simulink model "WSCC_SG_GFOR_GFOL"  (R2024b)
settings: Solver=ode1  StartTime=0.0  StopTime=sim_config.Tsim  RelTol=1e-3
undefined symbols (not defined in the file or in its folder): sim_config
libraries: myLibrary x24, spsThreePhaseVIMeasurementLib x12, spsPower3phInstantaneousLib x6, spspowerguiLib x1

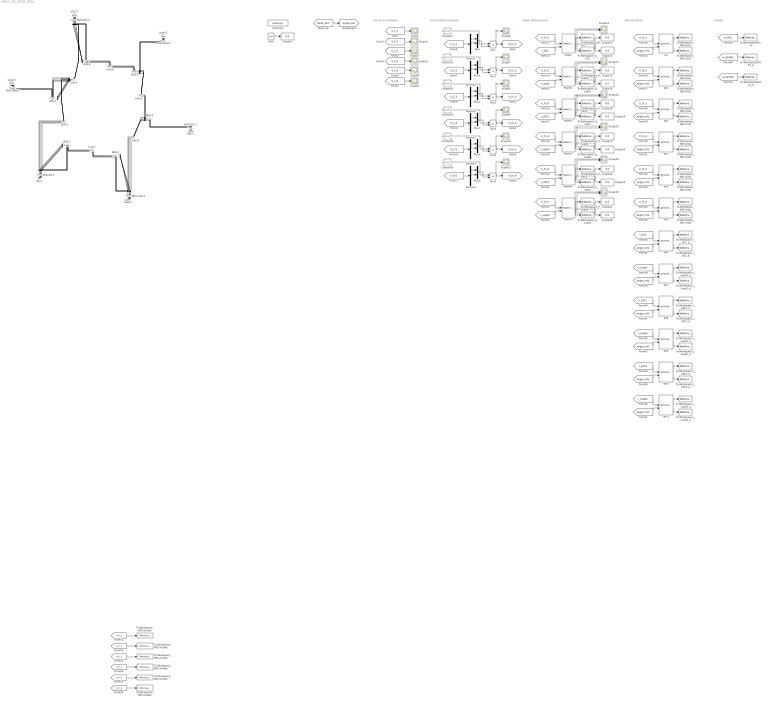
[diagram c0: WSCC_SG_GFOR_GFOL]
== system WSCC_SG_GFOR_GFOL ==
  note: Line-to-Line Voltages
  note: Line-to-Neutral Voltages
  note: Power Measurements
  note: qd0 transforms
  note: omega
  BUS-1 : spsThreePhaseVIMeasurementLib/Three-Phase V-I Measurement  VoltageMeasurement=phase-to-phase  SetLabelV=on  LabelV=V_ll_1  Vpu=off  VpuLL=off  CurrentMeasurement=yes  SetLabelI=on  LabelI=I_1  Ipu=off  Pbase=100e6  Vbase=500e3  OutputType=Complex  PhasorSimulation=off  PSBequivalent=0
  BUS-2 : spsThreePhaseVIMeasurementLib/Three-Phase V-I Measurement  VoltageMeasurement=phase-to-phase  SetLabelV=on  LabelV=V_ll_2  Vpu=off  VpuLL=off  CurrentMeasurement=yes  SetLabelI=on  LabelI=I_2  Ipu=off  Pbase=100e6  Vbase=500e3  OutputType=Complex  PhasorSimulation=off  PSBequivalent=0
  BUS-3 : spsThreePhaseVIMeasurementLib/Three-Phase V-I Measurement  VoltageMeasurement=phase-to-phase  SetLabelV=on  LabelV=V_ll_3  Vpu=off  VpuLL=off  CurrentMeasurement=yes  SetLabelI=on  LabelI=I_3  Ipu=off  Pbase=100e6  Vbase=500e3  OutputType=Complex  PhasorSimulation=off  PSBequivalent=0
  BUS-4 : spsThreePhaseVIMeasurementLib/Three-Phase V-I Measurement  VoltageMeasurement=phase-to-phase  SetLabelV=on  LabelV=V_ll_4  Vpu=off  VpuLL=off  CurrentMeasurement=yes  SetLabelI=on  LabelI=I_4  Ipu=off  Pbase=100e6  Vbase=500e3  OutputType=Complex  PhasorSimulation=off  PSBequivalent=0
  BUS-5 : spsThreePhaseVIMeasurementLib/Three-Phase V-I Measurement  VoltageMeasurement=phase-to-phase  SetLabelV=on  LabelV=V_ll_5  Vpu=off  VpuLL=off  CurrentMeasurement=yes  SetLabelI=on  LabelI=I_5  Ipu=off  Pbase=100e6  Vbase=500e3  OutputType=Complex  PhasorSimulation=off  PSBequivalent=0
  BUS-6 : spsThreePhaseVIMeasurementLib/Three-Phase V-I Measurement  VoltageMeasurement=phase-to-phase  SetLabelV=on  LabelV=V_ll_6  Vpu=off  VpuLL=off  CurrentMeasurement=yes  SetLabelI=on  LabelI=I_6  Ipu=off  Pbase=100e6  Vbase=500e3  OutputType=Complex  PhasorSimulation=off  PSBequivalent=0
  BUS-Load-1 : spsThreePhaseVIMeasurementLib/Three-Phase V-I Measurement  VoltageMeasurement=phase-to-phase  SetLabelV=on  LabelV=V_Load_1  Vpu=off  VpuLL=off  CurrentMeasurement=yes  SetLabelI=on  LabelI=I_Load1  Ipu=off  Pbase=100e6  Vbase=500e3  OutputType=Complex  PhasorSimulation=off  PSBequivalent=0
  BUS-Load-2 : spsThreePhaseVIMeasurementLib/Three-Phase V-I Measurement  VoltageMeasurement=phase-to-phase  SetLabelV=on  LabelV=V_Load_2  Vpu=off  VpuLL=off  CurrentMeasurement=yes  SetLabelI=on  LabelI=I_Load2  Ipu=off  Pbase=100e6  Vbase=500e3  OutputType=Complex  PhasorSimulation=off  PSBequivalent=0
  BUS-Load-3 : spsThreePhaseVIMeasurementLib/Three-Phase V-I Measurement  VoltageMeasurement=phase-to-phase  SetLabelV=on  LabelV=V_Load_3  Vpu=off  VpuLL=off  CurrentMeasurement=yes  SetLabelI=on  LabelI=I_Load3  Ipu=off  Pbase=100e6  Vbase=500e3  OutputType=Complex  PhasorSimulation=off  PSBequivalent=0
  BUS-SG-1 : spsThreePhaseVIMeasurementLib/Three-Phase V-I Measurement  VoltageMeasurement=phase-to-phase  SetLabelV=on  LabelV=V_SG_1  Vpu=off  VpuLL=off  CurrentMeasurement=yes  SetLabelI=on  LabelI=I_SG1  Ipu=off  Pbase=100e6  Vbase=500e3  OutputType=Complex  PhasorSimulation=off  PSBequivalent=0
  BUS-VSC-1 : spsThreePhaseVIMeasurementLib/Three-Phase V-I Measurement  VoltageMeasurement=phase-to-phase  SetLabelV=on  LabelV=V_VSC_1  Vpu=off  VpuLL=off  CurrentMeasurement=yes  SetLabelI=on  LabelI=I_VSC1  Ipu=off  Pbase=100e6  Vbase=500e3  OutputType=Complex  PhasorSimulation=off  PSBequivalent=0
  BUS-VSC-2 : spsThreePhaseVIMeasurementLib/Three-Phase V-I Measurement  VoltageMeasurement=phase-to-phase  SetLabelV=on  LabelV=V_VSC_2  Vpu=off  VpuLL=off  CurrentMeasurement=yes  SetLabelI=on  LabelI=I_VSC2  Ipu=off  Pbase=100e6  Vbase=500e3  OutputType=Complex  PhasorSimulation=off  PSBequivalent=0
  Constant{,1..5} (6 alike) : Constant  Value=[2/3 1/3; -1/3 1/3 ; -1/3 -2/3]
  Demux{,1..5} (6 alike) : Demux  Outputs=3
  Line-1 : myLibrary/PI_line  T_line_global=T_NET  initLine_global=init_line  num=1  set_C0=ones(1,6)  set_iL0=0
  Line-2 : myLibrary/PI_line  T_line_global=T_NET  initLine_global=init_line  num=2  set_C0="[1  0  0  1  1  1]"  set_iL0=0
  Line-3 : myLibrary/PI_line  T_line_global=T_NET  initLine_global=init_line  num=3  set_C0="[1  0  0  1  1  1]"  set_iL0=0
  Line-4 : myLibrary/PI_line  T_line_global=T_NET  initLine_global=init_line  num=4  set_C0="[1  0  0  1  1  1]"  set_iL0=0
  Line-5 : myLibrary/PI_line  T_line_global=T_NET  initLine_global=init_line  num=5  set_C0="[1  0  0  1  1  1]"  set_iL0=0
  Line-6 : myLibrary/PI_line  T_line_global=T_NET  initLine_global=init_line  num=6  set_C0=[1 0 0 1 0 0]  set_iL0=0
  Load-1 : myLibrary/Load_Rstep  T_load_global=T_load  initLoad_global=init_load  num=1  tstep=sim_config.tstep  Radd=Rload_add
  Load-2 : myLibrary/Load  T_load_global=T_load  initLoad_global=init_load  num=2
  Load-3 : myLibrary/Load  T_load_global=T_load  initLoad_global=init_load  num=3
  Mux{,1..5} (6 alike) : Mux  Inputs=2
  Power{,1..5} (6 alike) : spsPower3phInstantaneousLib/Power (3ph, Instantaneous)
  SG-1 : myLibrary/SG  num=1  init_SG_global=init_SG  initMachineBlocks=initMachineBlocks  T_SG_global=T_SG
  Scope{,1..11} (12 alike) : Scope
  Scope{12..13,15..16,18..19,21..22,24..25,27..28} (12 alike) : Display
  Scope{14,17,20,23,26,29} (6 alike) : Scope  NumInputPorts=2
  To WorkspaceGFOL2_w : ToWorkspace  VariableName=GFOL2_w  SampleTime=sim_config.Tsample
  To WorkspaceGFOR1_w : ToWorkspace  VariableName=GFOR1_w  SampleTime=sim_config.Tsample
  To WorkspaceSG1_w : ToWorkspace  VariableName=SG1_w  SampleTime=sim_config.Tsample
  To Workspace_I_Load1_d : ToWorkspace  VariableName=I_Load1_d  SampleTime=sim_config.Tsample
  To Workspace_I_Load1_q : ToWorkspace  VariableName=I_Load1_q  SampleTime=sim_config.Tsample
  To Workspace_I_Load2_d : ToWorkspace  VariableName=I_Load2_d  SampleTime=sim_config.Tsample
  To Workspace_I_Load2_q : ToWorkspace  VariableName=I_Load2_q  SampleTime=sim_config.Tsample
  To Workspace_I_Load3_d : ToWorkspace  VariableName=I_Load3_d  SampleTime=sim_config.Tsample
  To Workspace_I_Load3_q : ToWorkspace  VariableName=I_Load3_q  SampleTime=sim_config.Tsample
  To Workspace_I_SG1_d : ToWorkspace  VariableName=I_SG1_d  SampleTime=sim_config.Tsample
  To Workspace_I_SG1_q : ToWorkspace  VariableName=I_SG1_q  SampleTime=sim_config.Tsample
  To Workspace_I_VSC1_d : ToWorkspace  VariableName=I_VSC1_d  SampleTime=sim_config.Tsample
  To Workspace_I_VSC1_q : ToWorkspace  VariableName=I_VSC1_q  SampleTime=sim_config.Tsample
  To Workspace_I_VSC2_d : ToWorkspace  VariableName=I_VSC2_d  SampleTime=sim_config.Tsample
  To Workspace_I_VSC2_q : ToWorkspace  VariableName=I_VSC2_q  SampleTime=sim_config.Tsample
  To Workspace_NET.vn1abc : ToWorkspace  VariableName=vn1abc  SampleTime=sim_config.Tsample
  To Workspace_NET.vn1d : ToWorkspace  VariableName=vn1d  SampleTime=sim_config.Tsample
  To Workspace_NET.vn1q : ToWorkspace  VariableName=vn1q  SampleTime=sim_config.Tsample
  To Workspace_NET.vn2abc : ToWorkspace  VariableName=vn2abc  SampleTime=sim_config.Tsample
  To Workspace_NET.vn2d : ToWorkspace  VariableName=vn2d  SampleTime=sim_config.Tsample
  To Workspace_NET.vn2q : ToWorkspace  VariableName=vn2q  SampleTime=sim_config.Tsample
  To Workspace_NET.vn3abc : ToWorkspace  VariableName=vn3abc  SampleTime=sim_config.Tsample
  To Workspace_NET.vn3d : ToWorkspace  VariableName=vn3d  SampleTime=sim_config.Tsample
  To Workspace_NET.vn3q : ToWorkspace  VariableName=vn3q  SampleTime=sim_config.Tsample
  To Workspace_NET.vn4abc : ToWorkspace  VariableName=vn4abc  SampleTime=sim_config.Tsample
  To Workspace_NET.vn4d : ToWorkspace  VariableName=vn4d  SampleTime=sim_config.Tsample
  To Workspace_NET.vn4q : ToWorkspace  VariableName=vn4q  SampleTime=sim_config.Tsample
  To Workspace_NET.vn5abc : ToWorkspace  VariableName=vn5abc  SampleTime=sim_config.Tsample
  To Workspace_NET.vn5d : ToWorkspace  VariableName=vn5d  SampleTime=sim_config.Tsample
  To Workspace_NET.vn5q : ToWorkspace  VariableName=vn5q  SampleTime=sim_config.Tsample
  To Workspace_NET.vn6abc : ToWorkspace  VariableName=vn6abc  SampleTime=sim_config.Tsample
  To Workspace_NET.vn6d : ToWorkspace  VariableName=vn6d  SampleTime=sim_config.Tsample
  To Workspace_NET.vn6q : ToWorkspace  VariableName=vn6q  SampleTime=sim_config.Tsample
  To Workspace_P_Load1 : ToWorkspace  VariableName=P_Load1  SampleTime=sim_config.Tsample
  To Workspace_P_Load2 : ToWorkspace  VariableName=P_Load2  SampleTime=sim_config.Tsample
  To Workspace_P_Load3 : ToWorkspace  VariableName=P_Load3  SampleTime=sim_config.Tsample
  To Workspace_P_SG1 : ToWorkspace  VariableName=P_SG1  SampleTime=sim_config.Tsample
  To Workspace_P_VSC1 : ToWorkspace  VariableName=P_VSC1  SampleTime=sim_config.Tsample
  To Workspace_P_VSC2 : ToWorkspace  VariableName=P_VSC2  SampleTime=sim_config.Tsample
  To Workspace_Q_Load1 : ToWorkspace  VariableName=Q_Load1  SampleTime=sim_config.Tsample
  To Workspace_Q_Load2 : ToWorkspace  VariableName=Q_Load2  SampleTime=sim_config.Tsample
  To Workspace_Q_Load3 : ToWorkspace  VariableName=Q_Load3  SampleTime=sim_config.Tsample
  To Workspace_Q_SG1 : ToWorkspace  VariableName=Q_SG1  SampleTime=sim_config.Tsample
  To Workspace_Q_VSC1 : ToWorkspace  VariableName=Q_VSC1  SampleTime=sim_config.Tsample
  To Workspace_Q_VSC2 : ToWorkspace  VariableName=Q_VSC2  SampleTime=sim_config.Tsample
  VSC-1 : myLibrary/GFOR  T_VSC_global=T_VSC  initVSC_global=init_VSC  num=1
  VSC-2 : myLibrary/GFOL  T_VSC_global=T_VSC  initVSC_global=init_VSC  num=2
  clock : Clock
  display : Display
  mtx{,1..5} (6 alike) : Product  Multiplication=Matrix(*)
  powergui : spspowerguiLib/powergui  Priority=1  SimulationMode=Discrete  SampleTime=sim_config.Ts  frequency=60  Iterations=50  frequencyindice=50  Pbase=100e6  ErrMax=1e-4  UnitsV=kV  UnitsW=MW  buscounter=0  FunctionMessages=off  echomessages=off  EnableUseOfTLC=off  CurrentSourceSwitches=off  DisableSnubberDevices=off  DisableRonSwitches=off  DisableVfSwitches=off  DisplayEquations=off  AutomaticDiscreteSolvers=off  SolverType=Tustin/Backward Euler (TBE)  Interpol=off  ExternalGateDelay=off  methode=off  Ts=100  x0status=blocks  SPID=on  SwTol=0  HookPort=off  NonlinearTolerance=1e-4  nMaxIteration=100  ContinueOnMaxIteration=off  RestoreLinks=warning  ResistiveCurrentMeasurement=off  Frange=[0:2:500]  Ylog=off  Xlog=on  ShowGrid=off  save=off  variable=ZData  structure=0  ZoomFFT=off  StartTime=0.0  cycles=1  DisplayStyle=1  fundamental=60  FreqAxis=off  MaxFrequency=1000  frequencyindicesteady=1  RmsSteady=1  display=off
  qd{,1..11} (12 alike) : myLibrary/qd transform  SystemSampleTime=-1  VariantActivationTime=update diagram  AllowFlexibleInterface=on  Latency=0  AutoFrameSizeCalculation=off
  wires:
  clock/1 -> display/1
  [theta_SG1] -> [angle_ref1]
  [V_ll_1] -> Scope/1
  [V_ll_2] -> Scope1/1
  [V_ll_3] -> Scope2/1
  [V_ll_4] -> Scope3/1
  [V_ll_5] -> Scope4/1
  [V_ll_6] -> Scope5/1
  [V_ll_1] -> Demux/1
  Demux/1 -> Mux/1
  Demux/2 -> Mux/2
  Mux/1 -> mtx/2
  Constant/1 -> mtx/1
  mtx/1 -> [V_fn_1], Scope6/1
  [V_ll_2] -> Demux1/1
  Demux1/1 -> Mux1/1
  Demux1/2 -> Mux1/2
  Mux1/1 -> mtx1/2
  Constant1/1 -> mtx1/1
  mtx1/1 -> [V_fn_2], Scope7/1
  [V_ll_3] -> Demux2/1
  Demux2/1 -> Mux2/1
  Demux2/2 -> Mux2/2
  Mux2/1 -> mtx2/2
  Constant2/1 -> mtx2/1
  mtx2/1 -> [V_fn_3], Scope8/1
  [V_ll_4] -> Demux3/1
  Demux3/1 -> Mux3/1
  Demux3/2 -> Mux3/2
  Mux3/1 -> mtx3/2
  Constant3/1 -> mtx3/1
  mtx3/1 -> [V_fn_4], Scope9/1
  [V_ll_5] -> Demux4/1
  Demux4/1 -> Mux4/1
  Demux4/2 -> Mux4/2
  Mux4/1 -> mtx4/2
  Constant4/1 -> mtx4/1
  mtx4/1 -> [V_fn_5], Scope10/1
  [V_ll_6] -> Demux5/1
  Demux5/1 -> Mux5/1
  Demux5/2 -> Mux5/2
  Mux5/1 -> mtx5/2
  Constant5/1 -> mtx5/1
  mtx5/1 -> [V_fn_6], Scope11/1
  [V_fn_1] -> Power/1
  [I_SG1] -> Power/2
  Power/1 -> To Workspace_P_SG1/1, Scope12/1, Scope14/1
  Power/2 -> To Workspace_Q_SG1/1, Scope13/1, Scope14/2
  [V_fn_2] -> Power1/1
  [I_Load1] -> Power1/2
  Power1/1 -> To Workspace_P_Load1/1, Scope15/1, Scope17/1
  Power1/2 -> To Workspace_Q_Load1/1, Scope16/1, Scope17/2
  [V_fn_4] -> Power2/1
  [I_VSC1] -> Power2/2
  Power2/1 -> To Workspace_P_VSC1/1, Scope18/1, Scope20/1
  Power2/2 -> To Workspace_Q_VSC1/1, Scope19/1, Scope20/2
  [V_fn_3] -> Power3/1
  [I_Load2] -> Power3/2
  Power3/1 -> To Workspace_P_Load2/1, Scope21/1, Scope23/1
  Power3/2 -> To Workspace_Q_Load2/1, Scope22/1, Scope23/2
  [V_fn_6] -> Power4/1
  [I_VSC2] -> Power4/2
  Power4/1 -> To Workspace_P_VSC2/1, Scope24/1, Scope26/1
  Power4/2 -> To Workspace_Q_VSC2/1, Scope25/1, Scope26/2
  [V_fn_5] -> Power5/1
  [I_Load3] -> Power5/2
  Power5/1 -> To Workspace_P_Load3/1, Scope27/1, Scope29/1
  Power5/2 -> To Workspace_Q_Load3/1, Scope28/1, Scope29/2
  [V_fn_1] -> qd/1
  [angle_ref1] -> qd/2
  qd/1 -> To Workspace_NET.vn1q/1
  qd/2 -> To Workspace_NET.vn1d/1
  [V_fn_2] -> qd1/1
  [angle_ref1] -> qd1/2
  qd1/1 -> To Workspace_NET.vn2q/1
  qd1/2 -> To Workspace_NET.vn2d/1
  [V_fn_3] -> qd2/1
  [angle_ref1] -> qd2/2
  qd2/1 -> To Workspace_NET.vn3q/1
  qd2/2 -> To Workspace_NET.vn3d/1
  [V_fn_4] -> qd3/1
  [angle_ref1] -> qd3/2
  qd3/1 -> To Workspace_NET.vn4q/1
  qd3/2 -> To Workspace_NET.vn4d/1
  [V_fn_5] -> qd4/1
  [angle_ref1] -> qd4/2
  qd4/1 -> To Workspace_NET.vn5q/1
  qd4/2 -> To Workspace_NET.vn5d/1
  [V_fn_6] -> qd5/1
  [angle_ref1] -> qd5/2
  qd5/1 -> To Workspace_NET.vn6q/1
  qd5/2 -> To Workspace_NET.vn6d/1
  [I_SG1] -> qd6/1
  [angle_ref1] -> qd6/2
  qd6/1 -> To Workspace_I_SG1_q/1
  qd6/2 -> To Workspace_I_SG1_d/1
  [I_Load1] -> qd7/1
  [angle_ref1] -> qd7/2
  qd7/1 -> To Workspace_I_Load1_q/1
  qd7/2 -> To Workspace_I_Load1_d/1
  [I_VSC1] -> qd8/1
  [angle_ref1] -> qd8/2
  qd8/1 -> To Workspace_I_VSC1_q/1
  qd8/2 -> To Workspace_I_VSC1_d/1
  [I_Load2] -> qd9/1
  [angle_ref1] -> qd9/2
  qd9/1 -> To Workspace_I_Load2_q/1
  qd9/2 -> To Workspace_I_Load2_d/1
  [I_VSC2] -> qd10/1
  [angle_ref1] -> qd10/2
  qd10/1 -> To Workspace_I_VSC2_q/1
  qd10/2 -> To Workspace_I_VSC2_d/1
  [I_Load3] -> qd11/1
  [angle_ref1] -> qd11/2
  qd11/1 -> To Workspace_I_Load3_q/1
  qd11/2 -> To Workspace_I_Load3_d/1
  [w_SG1] -> To WorkspaceSG1_w/1
  [w_GFOR1] -> To WorkspaceGFOR1_w/1
  [w_GFOL2] -> To WorkspaceGFOL2_w/1
  [V_fn_1] -> To Workspace_NET.vn1abc/1
  [V_fn_2] -> To Workspace_NET.vn2abc/1
  [V_fn_3] -> To Workspace_NET.vn3abc/1
  [V_fn_4] -> To Workspace_NET.vn4abc/1
  [V_fn_5] -> To Workspace_NET.vn5abc/1
  [V_fn_6] -> To Workspace_NET.vn6abc/1
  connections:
  BUS-SG-1/RConn1 -- BUS-1/LConn1 -- Line-2/LConn1
  BUS-SG-1/RConn2 -- BUS-1/LConn2 -- Line-2/LConn2
  BUS-SG-1/RConn3 -- BUS-1/LConn3 -- Line-2/LConn3
  BUS-SG-1/LConn1 -- SG-1/RConn1
  BUS-SG-1/LConn2 -- SG-1/RConn2
  BUS-SG-1/LConn3 -- SG-1/RConn3
  BUS-1/RConn1 -- Line-1/LConn1
  BUS-1/RConn2 -- Line-1/LConn2
  BUS-1/RConn3 -- Line-1/LConn3
  Line-1/RConn1 -- BUS-2/LConn1
  Line-1/RConn2 -- BUS-2/LConn2
  Line-1/RConn3 -- BUS-2/LConn3
  BUS-Load-1/LConn1 -- BUS-2/RConn1 -- Line-3/LConn1
  BUS-Load-1/LConn2 -- BUS-2/RConn2 -- Line-3/LConn2
  BUS-Load-1/LConn3 -- BUS-2/RConn3 -- Line-3/LConn3
  BUS-Load-1/RConn1 -- Load-1/LConn1
  BUS-Load-1/RConn2 -- Load-1/LConn2
  BUS-Load-1/RConn3 -- Load-1/LConn3
  BUS-4/LConn1 -- Line-3/RConn1 -- Line-5/LConn1
  BUS-4/LConn2 -- Line-3/RConn2 -- Line-5/LConn2
  BUS-4/LConn3 -- Line-3/RConn3 -- Line-5/LConn3
  BUS-4/RConn1 -- BUS-VSC-1/RConn1
  BUS-4/RConn2 -- BUS-VSC-1/RConn2
  BUS-4/RConn3 -- BUS-VSC-1/RConn3
  BUS-VSC-1/LConn1 -- VSC-1/RConn1
  BUS-VSC-1/LConn2 -- VSC-1/RConn2
  BUS-VSC-1/LConn3 -- VSC-1/RConn3
  BUS-5/RConn1 -- Line-5/RConn1 -- BUS-Load-3/LConn1
  BUS-5/RConn2 -- Line-5/RConn2 -- BUS-Load-3/LConn2
  BUS-5/RConn3 -- Line-5/RConn3 -- BUS-Load-3/LConn3
  BUS-Load-3/RConn1 -- Load-3/LConn1
  BUS-Load-3/RConn2 -- Load-3/LConn2
  BUS-Load-3/RConn3 -- Load-3/LConn3
  BUS-5/LConn1 -- Line-6/LConn1
  BUS-5/LConn2 -- Line-6/LConn2
  BUS-5/LConn3 -- Line-6/LConn3
  Line-6/RConn1 -- BUS-6/RConn1
  Line-6/RConn2 -- BUS-6/RConn2
  Line-6/RConn3 -- BUS-6/RConn3
  BUS-VSC-2/RConn1 -- BUS-6/LConn1 -- Line-4/RConn1
  BUS-VSC-2/RConn2 -- BUS-6/LConn2 -- Line-4/RConn2
  BUS-VSC-2/RConn3 -- BUS-6/LConn3 -- Line-4/RConn3
  BUS-VSC-2/LConn1 -- VSC-2/RConn1
  BUS-VSC-2/LConn2 -- VSC-2/RConn2
  BUS-VSC-2/LConn3 -- VSC-2/RConn3
  Line-4/LConn1 -- BUS-3/RConn1 -- Line-2/RConn1
  Line-4/LConn2 -- BUS-3/RConn2 -- Line-2/RConn2
  Line-4/LConn3 -- BUS-3/RConn3 -- Line-2/RConn3
  BUS-3/LConn1 -- BUS-Load-2/LConn1
  BUS-3/LConn2 -- BUS-Load-2/LConn2
  BUS-3/LConn3 -- BUS-Load-2/LConn3
  BUS-Load-2/RConn1 -- Load-2/LConn1
  BUS-Load-2/RConn2 -- Load-2/LConn2
  BUS-Load-2/RConn3 -- Load-2/LConn3
